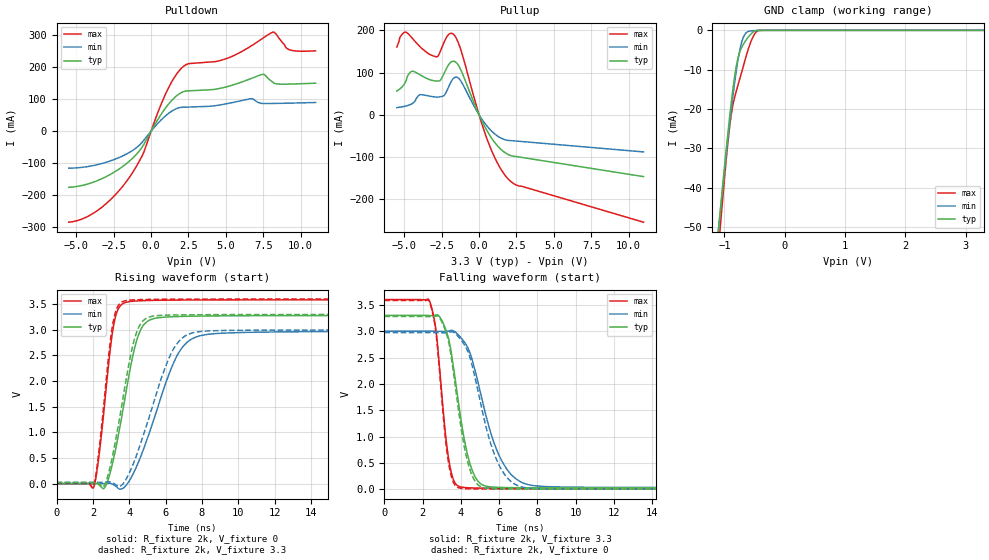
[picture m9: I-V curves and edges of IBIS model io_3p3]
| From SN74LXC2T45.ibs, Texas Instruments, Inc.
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[Model]   io_3p3
Model_type  I/O
Vinl=0.8
Vinh=2.0
Enable   Active-Low
Vref =   0
Rref =   2000
Cref =   15p
Vmeas =   1.5
| variable   typ   min   max
C_comp   6.05pF   5.21pF   7.21pF
| C_pullup   14.02pF   6.09pF   25.42pF
| C_pulldown   9.23pF   6.55pF   14.97pF
| C_tri-state   6.05pF   5.21pF   7.21pF
[Temperature Range]   40   100   -40
| Ambient temperature   25   85   -40
[Voltage range]   3.3   3   3.6
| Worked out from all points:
|   slope of the pulldown table from 0 to 0.495 V, typ, clamps not added: 12.4 ohm
|   slope of the pullup table from 0 to 0.495 V, typ, clamps not added: 14 ohm
|   GND clamp passes 1 mA (typ) near -0.56 V on its own axis
|   rising waveform, R_fixture 2k, V_fixture 0: 20-80 % time 1.04ns typ, 1.77ns min, 650ps max; typ from 0 V to 3.28 V
|   falling waveform, R_fixture 2k, V_fixture 3.3: 20-80 % time 862ps typ, 1.4ns min, 560ps max; typ from 3.3 V to 0.019 V
|   rising waveform, R_fixture 2k, V_fixture 3.3: 20-80 % time 1.01ns typ, 1.67ns min, 635ps max; typ from 0.019 V to 3.3 V
|   falling waveform, R_fixture 2k, V_fixture 0: 20-80 % time 817ps typ, 1.26ns min, 542ps max; typ from 3.28 V to 0 V
[GND Clamp]
| LXC8T245_IO_33
|   Voltage   I(typ)   I(min)   I(max)
-5.5V     -897.1mA   -831.9mA   -1.015A
-1.095V   -50.17mA   -50.04mA   -54.92mA
-1.065V   -45.25mA   -45.49mA   -49.39mA
-970mV    -30.27mA   -31.55mA   -32.88mA
-905mV    -20.84mA   -22.59mA   -23.49mA
-860mV    -15.02mA   -16.81mA   -19.04mA
-790mV    -8.096mA   -8.927mA   -14.74mA
-735mV    -5.102mA   -4.277mA   -11.79mA
-675mV    -3.272mA   -1.404mA   -8.498mA
-560mV    -930.2uA   -146.6uA   -2.855mA
-455mV    -11.08uA   -48.45uA   -188.9uA
3.3V      32.42pA    190.2nA    586.5pA
[Pulldown]
| LXC8T245_IO_33
|   Voltage   I(typ)   I(min)   I(max)
-5.5V     -176.2mA   -116.1mA   -285.6mA
-3.56V    -154.7mA   -104.8mA   -248.1mA
-1.62V    -100.7mA   -71.19mA   -156.1mA
-535mV    -45.52mA   -31.12mA   -71.38mA
1.155V    84.06mA    55.16mA    134.7mA
2.23V     124.7mA    75.07mA    205.2mA
5.1V      139.6mA    86.34mA    228.5mA
6.75V     166.1mA    101.8mA    268.8mA
7.495V    178.1mA    86.65mA    292mA
8.17V     152.3mA    86.77mA    310.5mA
9.2V      147.4mA    87.68mA    256mA
11V       150.3mA    89.74mA    251.8mA
[Pullup]
| LXC8T245_IO_33
|   Voltage   I(typ)   I(min)   I(max)
-5.5V     56.18mA    16.98mA    160.3mA
-4.89V    79.66mA    20.64mA    195.7mA
-4.445V   103.3mA    26.89mA    180.5mA
-3.945V   94.62mA    47.4mA     161.1mA
-2.805V   79.84mA    41.85mA    137.4mA
-2.095V   114.9mA    61.02mA    187.6mA
-1.66V    126.5mA    87.57mA    189.1mA
-1.24V    108mA      81.18mA    156.3mA
695mV     -47.39mA   -33.41mA   -72.26mA
1.475V    -82.35mA   -55.39mA   -129.6mA
2.255V    -98mA      -61.58mA   -161.7mA
11V       -146.5mA   -88.02mA   -254.5mA
[Ramp]
| LXC8T245_IO_33
| variable   typ   min   max
dV/dt_r   1.98/0.66E-09   1.78/0.95E-09   2.17/8.51E-10
dV/dt_f   1.98/7.52E-10   1.78/1.2E-09   2.17/6.07E-10
R_load = 2k
[Rising Waveform]
| LXC8T245_IO_33
R_fixture =   2k
C_fixture =   0
L_fixture =   0
V_fixture =   0
V_fixture_min = 0
V_fixture_max = 0
|   Time   V(typ)   V(min)   V(max)
0s        346pV      6.356nV    1.892nV
2.055ns   1.068mV    -1.68uV    -61.68mV
2.61ns    -93.84mV   118.6uV    1.428V
3.125ns   464.3mV    -18.53mV   3.053V
3.82ns    1.781V     -36.42mV   3.536V
4.36ns    2.732V     298.2mV    3.562V
4.865ns   3.125V     749.2mV    3.57V
6.595ns   3.258V     2.473V     3.58V
7.86ns    3.268V     2.881V     3.582V
34.99ns   3.279V     2.973V     3.584V
[Falling Waveform]
| LXC8T245_IO_33
R_fixture =   2k
C_fixture =   0
L_fixture =   0
V_fixture =   3.3
V_fixture_min = 3
V_fixture_max = 3.6
|   Time   V(typ)   V(min)   V(max)
0s        3.3V       3V         3.6V
2.365ns   3.298V     3V         3.566V
2.705ns   3.309V     2.999V     2.98V
3.37ns    2.833V     3.005V     543mV
3.95ns    1.442V     2.896V     45.68mV
4.42ns    548.6mV    2.637V     25.86mV
4.92ns    139.1mV    1.986V     21mV
6.065ns   33.13mV    588.5mV    18mV
7.49ns    25.65mV    88.17mV    15.96mV
34.99ns   19.26mV    26.22mV    13.14mV
[Rising Waveform]
| LXC8T245_IO_33
R_fixture =   2k
C_fixture =   0
L_fixture =   0
V_fixture =   3.3
V_fixture_min = 3
V_fixture_max = 3.6
|   Time   V(typ)   V(min)   V(max)
0s        19.2mV     25.88mV    13.13mV
2.04ns    19.86mV    25.88mV    -41.85mV
2.6ns     -52.64mV   25.93mV    1.537V
3.075ns   530.8mV    17.65mV    3.068V
3.735ns   1.837V     33.43mV    3.562V
4.255ns   2.778V     416.3mV    3.585V
4.73ns    3.165V     893.1mV    3.59V
6.29ns    3.288V     2.53V      3.597V
7.48ns    3.294V     2.94V      3.598V
34.99ns   3.3V       3V         3.6V
[Falling Waveform]
| LXC8T245_IO_33
R_fixture =   2k
C_fixture =   0
L_fixture =   0
V_fixture =   0
V_fixture_min = 0
V_fixture_max = 0
|   Time   V(typ)   V(min)   V(max)
0s        3.279V     2.974V     3.585V
2.36ns    3.277V     2.974V     3.553V
2.695ns   3.287V     2.973V     2.966V
3.345ns   2.816V     2.977V     515.5mV
3.9ns     1.428V     2.881V     24.34mV
4.345ns   525.8mV    2.631V     7.26mV
4.82ns    110mV      1.985V     4.059mV
5.885ns   6.085mV    541.1mV    2.961mV
7.19ns    2.345mV    40.66mV    1.88mV
34.99ns   58.97uV    216uV      7.446uV
